| IBIS file generated by GenIBIS.pl Version 3.10
|   netra
[IBIS ver]   4.1
[File name]   DM816x.ibs
[File Rev]   1.0
[Date]   Wed Jul 14, 2010, 9:28:38
[Source]   Data created at Texas Instruments
[Notes]   Checked with IBISCHK4 : 16 warnings
   3 warnings relating to single model selectors should be waived
   13 warning relating to max data is non-monotonic should be waived
[Disclaimer] Please be aware that in the absence of a written agreement,
   Texas Instruments (TI) assumes no liability for: 1) the
   accuracy of the IBIS models provided to your company, 2) the
   proper functioning of these IBIS models in your design or for
   any resulting applications, or, 3) infringement of patents,
   copyrights, or intellectual property rights resulting from
   your use of these IBIS models. TI provides IBIS models as a
   service to our customers and therefore reserves the right to
   limit distribution of the IBIS models.
[Copyright]   Property of Texas Instruments Incorporated. Unauthorised
   reproduction and/or distribution is strictly prohibited. This
   product is protected under copyright law and trade secret law
   as an unpublished work. Created 2010,(C) Copyright 2010,
   Texas Instruments Incorporated., All Rights Reserved. These
   commodities are under the U.S. Government distribution license
   control.As such,they are not to be re-exported without the
   prior approval of the U.S. Department of Commerce.
|   Component netra
[Component]   netra
[Manufacturer]   Texas Instruments.
[Package]
|   typ   min   max
R_pkg   1083.455m   49.41m   2117.50m
L_pkg   3.26nH   0.72nH   5.80nH
C_pkg   1.9pF   0.63pF   3.17pF
[Pin]   signal_name   model_name   R_pin   L_pin   C_pin
H37   CLKIN32   Selector_1   1309.20m   3.65nH   1.83pF
F1   CLKOUT   Selector_1   1491.00m   3.78nH   1.94pF
C9   DDR0_D31   Selector_4   1469.70m   3.53nH   1.82pF
C18   DDR0_CKE   Selector_2   1358.20m   3.54nH   1.63pF
B10   DDR0_D26   Selector_4   1460.70m   3.63nH   1.97pF
D2   DDR0_D4   Selector_4   1531.00m   3.98nH   2.12pF
F2   DDR0_D1   Selector_4   1518.50m   3.74nH   2.08pF
C11   DDR0_D29   Selector_4   1449.60m   3.76nH   1.97pF
E18   DDR0_ODT0   Selector_2   1256.70m   3.57nH   1.67pF
A14   DDR0_A7   Selector_2   1331.60m   3.52nH   1.86pF
D7   DDR0_D9   Selector_4   1744.10m   4.10nH   2.16pF
C13   DDR0_CASN   Selector_2   1332.10m   3.61nH   1.86pF
C8   DDR0_D16   Selector_4   1423.40m   3.34nH   1.91pF
G10   DDR0_D28   Selector_4   1486.50m   3.61nH   2.07pF
F13   DDR0_BA0   Selector_2   1260.70m   3.24nH   1.75pF
L13   DDR0_A6   Selector_2   1153.10m   3.02nH   1.61pF
E13   DDR0_WEN   Selector_2   1287.90m   3.35nH   1.78pF
B13   DDR0_A11   Selector_2   1352.50m   3.67nH   1.95pF
D8   DDR0_D21   Selector_4   1394.50m   3.33nH   2.05pF
B12   DDR0_CLK0   Selector_2   1415.20m   3.69nH   1.69pF
C2   DDR0_DQM0   Selector_2   1527.40m   3.89nH   2.14pF
A16   DDR0_ODT1   Selector_2   1375.80m   3.74nH   1.86pF
B14   DDR0_BA1   Selector_2   1319.50m   3.63nH   1.86pF
K13   DDR0_A9   Selector_2   1252.40m   3.22nH   1.70pF
B7   DDR0_D19   Selector_4   1383.00m   3.34nH   1.95pF
B16   DDR0_A13   Selector_2   1270.10m   3.37nH   1.81pF
B6   DDR0_D13   Selector_4   1710.40m   4.12nH   2.18pF
D18   DDR0_RST   Selector_2   1315.90m   3.41nH   1.71pF
E3   DDR0_DQSN0   Selector_7   1601.30m   3.84nH   1.94pF
N14   DDR0_A8   Selector_2   1151.50m   3.06nH   1.57pF
B17   DDR0_CSN0   Selector_2   1349.40m   3.49nH   1.72pF
H10   DDR0_D18   Selector_4   1427.20m   3.35nH   2.06pF
A3   DDR0_D14   Selector_4   1766.10m   4.41nH   2.34pF
A5   DDR0_D12   Selector_4   1740.90m   4.25nH   2.37pF
A12   DDR0_CLK0N   Selector_2   1403.00m   3.48nH   1.71pF
E2   DDR0_D2   Selector_4   1529.70m   3.83nH   2.00pF
C1   DDR0_D7   Selector_4   1537.70m   3.99nH   2.06pF
N15   DDR0_BA2   Selector_2   1133.30m   3.22nH   1.44pF
B3   DDR0_D15   Selector_4   1746.20m   4.07nH   2.26pF
A9   DDR0_DQSN3   Selector_7   1585.40m   3.85nH   1.84pF
N16   DDR0_A12   Selector_2   1122.70m   3.13nH   1.44pF
C14   DDR0_A10   Selector_2   1298.30m   3.51nH   1.79pF
F3   DDR0_D6   Selector_4   1543.60m   4.02nH   2.09pF
B2   DDR0_D5   Selector_4   1489.90m   3.72nH   2.04pF
A8   DDR0_DQSN2   Selector_7   1538.30m   3.73nH   1.90pF
B9   DDR0_DQS3   Selector_7   1600.40m   3.82nH   1.84pF
B5   DDR0_DQM1   Selector_2   1739.40m   4.39nH   2.24pF
E8   DDR0_D27   Selector_4   1430.00m   3.59nH   1.99pF
J11   DDR0_D30   Selector_4   1504.00m   3.69nH   1.90pF
J13   DDR0_A5   Selector_2   1333.50m   3.39nH   1.68pF
E7   DDR0_D23   Selector_4   1403.30m   3.52nH   1.96pF
A13   DDR0_A0   Selector_2   1265.50m   3.65nH   1.74pF
A15   DDR0_CLK1   Selector_2   1409.10m   3.47nH   1.71pF
A4   DDR0_DQSN1   Selector_7   1881.10m   4.39nH   2.13pF
G4   DDR0_D3   Selector_4   1490.40m   3.74nH   2.07pF
B8   DDR0_DQS2   Selector_7   1535.10m   3.81nH   1.76pF
A7   DDR0_D17   Selector_4   1476.50m   3.78nH   1.93pF
B4   DDR0_DQS1   Selector_7   1878.40m   4.27nH   2.13pF
D17   DDR0_A14   Selector_2   1253.70m   3.19nH   1.81pF
C6   DDR0_D10   Selector_4   1782.00m   4.37nH   2.22pF
H13   DDR0_A4   Selector_2   1256.10m   3.18nH   1.74pF
E9   DDR0_D24   Selector_4   1434.50m   3.63nH   1.86pF
D9   DDR0_DQM3   Selector_2   1479.60m   3.74nH   1.92pF
D13   DDR0_RASN   Selector_2   1266.70m   3.18nH   1.82pF
B1   DDR0_D0   Selector_4   1470.70m   3.76nH   2.13pF
C5   DDR0_D8   Selector_4   1688.70m   3.78nH   2.09pF
N17   DDR0_A1   Selector_2   1196.40m   3.20nH   1.58pF
F8   DDR0_D20   Selector_4   1427.80m   3.64nH   1.98pF
F9   DDR0_D22   Selector_4   1439.50m   3.61nH   1.90pF
D6   DDR0_D11   Selector_4   1736.00m   3.98nH   2.27pF
G9   DDR0_DQM2   Selector_2   1448.90m   3.58nH   1.95pF
F4   DDR0_DQS0   Selector_7   1620.50m   3.95nH   1.97pF
F18   DDR0_CSN1   Selector_2   1308.20m   3.34nH   1.73pF
D15   DDR0_A2   Selector_2   1293.60m   3.44nH   1.80pF
G13   DDR0_A3   Selector_2   1313.50m   3.47nH   1.69pF
B15   DDR0_CLK1N   Selector_2   1400.90m   3.42nH   1.71pF
B11   DDR0_D25   Selector_4   1487.80m   3.56nH   1.92pF
F36   DDR1_D1   Selector_4   1516.50m   3.72nH   2.10pF
K25   DDR1_A9   Selector_2   1252.70m   3.22nH   1.71pF
B27   DDR1_D25   Selector_4   1494.60m   3.90nH   1.92pF
A35   DDR1_D14   Selector_4   1761.50m   4.48nH   2.31pF
E35   DDR1_DQSN0   Selector_7   1600.60m   3.84nH   1.86pF
L25   DDR1_A6   Selector_2   1146.20m   2.92nH   1.59pF
G34   DDR1_D3   Selector_4   1489.80m   3.78nH   2.08pF
B32   DDR1_D13   Selector_4   1708.80m   4.35nH   2.32pF
C20   DDR1_CKE   Selector_2   1327.50m   3.43nH   1.63pF
C24   DDR1_A10   Selector_2   1281.10m   3.40nH   1.81pF
D20   DDR1_RST   Selector_2   1302.90m   3.49nH   1.67pF
C29   DDR1_D31   Selector_4   1476.80m   3.76nH   1.94pF
E29   DDR1_D24   Selector_4   1437.50m   3.70nH   1.97pF
B22   DDR1_A13   Selector_2   1250.70m   3.43nH   1.78pF
C33   DDR1_D8   Selector_4   1686.90m   4.14nH   2.13pF
B31   DDR1_D19   Selector_4   1383.90m   3.59nH   1.84pF
C37   DDR1_D7   Selector_4   1538.40m   3.97nH   2.11pF
B33   DDR1_DQM1   Selector_2   1739.30m   4.30nH   2.28pF
E36   DDR1_D2   Selector_4   1529.70m   3.92nH   2.08pF
F20   DDR1_CSN1   Selector_2   1298.80m   3.39nH   1.72pF
D25   DDR1_RASN   Selector_2   1251.90m   3.31nH   1.80pF
C36   DDR1_DQM0   Selector_2   1526.50m   4.01nH   2.09pF
N22   DDR1_A12   Selector_2   1129.60m   3.36nH   1.44pF
N24   DDR1_A8   Selector_2   1151.30m   3.03nH   1.54pF
B21   DDR1_CSN0   Selector_2   1338.00m   3.57nH   1.74pF
B36   DDR1_D5   Selector_4   1496.60m   3.79nH   2.09pF
N21   DDR1_A1   Selector_2   1193.70m   3.19nH   1.60pF
F30   DDR1_D20   Selector_4   1426.70m   3.75nH   1.94pF
E30   DDR1_D27   Selector_4   1425.40m   3.68nH   2.08pF
C30   DDR1_D16   Selector_4   1420.60m   3.50nH   2.00pF
A34   DDR1_DQSN1   Selector_7   1885.10m   4.38nH   2.14pF
B28   DDR1_D26   Selector_4   1457.10m   3.72nH   1.90pF
A25   DDR1_A0   Selector_2   1266.80m   3.73nH   1.79pF
J27   DDR1_D30   Selector_4   1507.60m   3.72nH   2.06pF
A26   DDR1_CLK0N   Selector_2   1408.90m   3.58nH   1.67pF
B37   DDR1_D0   Selector_4   1469.70m   3.83nH   2.00pF
F35   DDR1_D6   Selector_4   1543.90m   3.99nH   2.08pF
N23   DDR1_BA2   Selector_2   1141.30m   3.31nH   1.43pF
B26   DDR1_CLK0   Selector_2   1421.50m   3.73nH   1.56pF
E20   DDR1_ODT0   Selector_2   1246.60m   3.51nH   1.69pF
B25   DDR1_A11   Selector_2   1335.80m   3.85nH   1.84pF
D21   DDR1_A14   Selector_2   1262.30m   3.15nH   1.77pF
B30   DDR1_DQS2   Selector_7   1543.40m   3.74nH   1.70pF
A31   DDR1_D17   Selector_4   1477.60m   3.79nH   1.89pF
E31   DDR1_D23   Selector_4   1404.30m   3.60nH   2.03pF
C27   DDR1_D29   Selector_4   1448.30m   3.80nH   2.01pF
A29   DDR1_DQSN3   Selector_7   1598.60m   3.83nH   1.94pF
J25   DDR1_A5   Selector_2   1309.60m   3.41nH   1.73pF
G29   DDR1_DQM2   Selector_2   1449.00m   3.60nH   1.92pF
D29   DDR1_DQM3   Selector_2   1482.20m   3.81nH   2.01pF
C25   DDR1_CASN   Selector_2   1319.50m   3.60nH   1.85pF
A22   DDR1_ODT1   Selector_2   1360.60m   3.61nH   1.87pF
E25   DDR1_WEN   Selector_2   1267.60m   3.39nH   1.80pF
A30   DDR1_DQSN2   Selector_7   1544.90m   3.83nH   1.76pF
D32   DDR1_D11   Selector_4   1733.00m   4.16nH   2.21pF
F34   DDR1_DQS0   Selector_7   1622.30m   3.89nH   1.76pF
B29   DDR1_DQS3   Selector_7   1607.10m   4.02nH   1.86pF
A33   DDR1_D12   Selector_4   1736.90m   4.33nH   2.28pF
D31   DDR1_D9   Selector_4   1747.90m   4.19nH   2.19pF
A24   DDR1_A7   Selector_2   1317.50m   3.61nH   1.88pF
H25   DDR1_A4   Selector_2   1241.80m   3.15nH   1.69pF
G28   DDR1_D28   Selector_4   1477.50m   3.63nH   2.05pF
D36   DDR1_D4   Selector_4   1532.20m   3.94nH   2.16pF
G25   DDR1_A3   Selector_2   1301.50m   3.47nH   1.74pF
B24   DDR1_BA1   Selector_2   1300.70m   3.55nH   1.82pF
D30   DDR1_D21   Selector_4   1394.40m   3.59nH   1.98pF
D23   DDR1_A2   Selector_2   1279.00m   3.38nH   1.87pF
F25   DDR1_BA0   Selector_2   1249.40m   3.21nH   1.71pF
H28   DDR1_D18   Selector_4   1427.50m   3.48nH   1.90pF
B35   DDR1_D15   Selector_4   1754.70m   4.28nH   2.24pF
F29   DDR1_D22   Selector_4   1441.70m   3.68nH   1.89pF
A23   DDR1_CLK1   Selector_2   1408.60m   3.54nH   1.77pF
C32   DDR1_D10   Selector_4   1784.80m   4.48nH   2.18pF
B34   DDR1_DQS1   Selector_7   1881.40m   4.41nH   2.08pF
B23   DDR1_CLK1N   Selector_2   1400.10m   3.58nH   1.69pF
J35   EMU0   Selector_3   1645.80m   4.47nH   2.22pF
L36   EMU1   Selector_3   1287.90m   3.82nH   1.76pF
L37   EMU2   Selector_3   1334.20m   3.65nH   1.85pF
M36   EMU3   Selector_3   1079.80m   3.03nH   1.65pF
M37   EMU4   Selector_3   1302.60m   3.45nH   1.77pF
AG28   GMII0_TXD4   Selector_3   564.85m   1.69nH   1.08pF
AE34   GMII0_RXER   Selector_3   916.91m   2.56nH   1.42pF
AF36   GMII0_TXD5   Selector_3   1240.00m   3.21nH   1.63pF
AF37   GMII0_TXCLK   Selector_3   1350.00m   3.67nH   1.87pF
AD25   GMII0_RXD5   Selector_3   170.60m   1.01nH   0.78pF
AE36   GMII0_RXD7   Selector_3   1288.30m   3.53nH   1.68pF
AE30   GMII0_TXD3   Selector_3   493.69m   1.61nH   1.01pF
AE33   GMII0_TXD0   Selector_3   986.48m   2.66nH   1.40pF
AE37   GMII0_RXCLK   Selector_3   1509.90m   3.89nH   2.04pF
AE32   GMII0_TXD1   Selector_3   762.14m   2.22nH   1.20pF
AG35   GMII0_TXD7   Selector_3   1051.50m   2.91nH   1.59pF
AC35   GMII0_RXD4   Selector_3   1124.40m   3.09nH   1.69pF
AC25   GMII0_RXD6   Selector_3   92.81m   0.81nH   0.65pF
AE31   GMII0_TXD2   Selector_3   828.93m   2.29nH   1.22pF
AG36   GMII0_TXD6   Selector_3   1331.80m   3.61nH   1.78pF
AD35   GMII0_RXD3   Selector_3   947.25m   2.61nH   1.46pF
AD37   GMII0_RXD0   Selector_3   1306.50m   3.47nH   1.77pF
AD36   GMII0_RXD1   Selector_3   1427.60m   3.90nH   1.76pF
AA25   GMII0_CRS   Selector_3   100.59m   0.85nH   0.71pF
AC37   GMII0_GTXCLK   Selector_3   1221.60m   3.13nH   1.69pF
AG37   GMII0_TXEN   Selector_3   1452.10m   3.88nH   1.95pF
AB25   GMII0_COL   Selector_3   226.60m   1.06nH   0.71pF
AE35   GMII0_RXDV   Selector_3   1056.10m   2.91nH   1.55pF
AC36   GMII0_RXD2   Selector_3   1200.10m   3.19nH   1.70pF
K31   GP0_IO0   Selector_1   795.97m   2.24nH   1.35pF
G5   GP0_IO6   Selector_1   1196.30m   3.27nH   1.74pF
G2   GP0_IO5   Selector_1   1205.80m   3.58nH   1.79pF
H32   GP0_IO4   Selector_1   1092.10m   2.82nH   1.67pF
H35   GP0_IO7   Selector_1   1083.40m   3.13nH   1.75pF
K30   GP0_IO2   Selector_1   925.22m   2.65nH   1.41pF
L29   GP0_IO1   Selector_1   694.30m   2.11nH   1.26pF
J31   GP0_IO3   Selector_1   1017.90m   2.83nH   1.55pF
J33   GP1_IO31   Selector_1   1137.80m   3.33nH   1.68pF
J32   GP1_IO30   Selector_1   1020.50m   2.79nH   1.56pF
AA3   GPMC_D3   Selector_1   1056.40m   2.99nH   1.56pF
AE1   GPMC_A4   Selector_1   1377.50m   3.92nH   1.90pF
AD3   GPMC_A7   Selector_1   1196.70m   3.32nH   1.73pF
W3   GPMC_D10   Selector_1   1112.50m   3.04nH   1.53pF
Y10   GPMC_D6   Selector_1   352.48m   1.25nH   0.89pF
AD1   GPMC_A10   Selector_1   1395.90m   3.72nH   1.87pF
Y3   GPMC_D4   Selector_1   1143.00m   3.16nH   1.62pF
AD8   GPMC_A6   Selector_1   1530.30m   4.11nH   2.05pF
AG3   GPMC_CS4   Selector_1   1297.50m   3.69nH   1.80pF
W2   GPMC_D12   Selector_1   966.20m   2.79nH   1.53pF
AC2   GPMC_A11   Selector_1   1362.40m   3.66nH   1.85pF
AC1   GPMC_D0   Selector_1   1233.50m   3.39nH   1.85pF
AA2   GPMC_D5   Selector_1   1118.40m   3.28nH   1.58pF
AE2   GPMC_A5   Selector_1   1495.60m   3.99nH   1.96pF
V1   GPMC_CLK   Selector_1   1272.40m   3.48nH   1.79pF
AG2   GPMC_WEN   Selector_1   1545.10m   4.10nH   2.08pF
V10   GPMC_D13   Selector_1   184.75m   0.89nH   0.73pF
AE4   GPMC_A2   Selector_1   1235.40m   3.43nH   1.67pF
AA4   GPMC_D1   Selector_1   1051.20m   2.95nH   1.51pF
AH7   GPMC_CS0   Selector_1   1189.60m   3.37nH   1.71pF
Y1   GPMC_D9   Selector_1   1157.00m   3.26nH   1.75pF
AH1   GPMC_CS1   Selector_1   1653.70m   4.70nH   2.01pF
AE10   GPMC_ADVN_ALE   Selector_1   1720.10m   4.77nH   2.21pF
AD4   GPMC_A8   Selector_1   1152.80m   3.26nH   1.73pF
AE7   GPMC_DIR   Selector_1   1320.10m   3.72nH   1.87pF
AE3   GPMC_A3   Selector_1   1358.60m   3.79nH   1.85pF
AF2   GPMC_OEN_REN   Selector_1   1476.20m   3.88nH   1.94pF
AH2   GPMC_CS2   Selector_1   1411.50m   3.83nH   2.11pF
AG1   GPMC_CS5   Selector_1   1663.40m   4.38nH   2.09pF
Y2   GPMC_D7   Selector_1   1171.80m   3.24nH   1.63pF
W1   GPMC_D11   Selector_1   1141.60m   3.23nH   1.64pF
W4   GPMC_D8   Selector_1   980.65m   2.85nH   1.47pF
AE11   GPMC_BE0N_CLE   Selector_1   532.49m   1.84nH   1.17pF
V2   GPMC_D15   Selector_1   1141.50m   3.10nH   1.63pF
AF1   GPMC_BE1N   Selector_1   1416.40m   3.85nH   2.00pF
AD2   GPMC_A9   Selector_1   1429.00m   3.83nH   1.94pF
AE9   GPMC_WPN   Selector_1   1318.70m   3.47nH   1.88pF
AE6   GPMC_A0   Selector_1   1350.00m   3.73nH   2.00pF
V3   GPMC_D14   Selector_1   1008.30m   2.79nH   1.47pF
AG9   GPMC_CS3   Selector_1   1366.30m   3.85nH   2.05pF
AC5   GPMC_A27   Selector_1   1270.00m   3.50nH   1.93pF
AE8   GPMC_WAIT   Selector_1   1441.30m   4.00nH   1.90pF
AB2   GPMC_D2   Selector_1   1290.40m   3.51nH   1.73pF
AE5   GPMC_A1   Selector_1   1097.80m   3.10nH   1.66pF
AE24   HDMI_HPDET   Selector_1   316.48m   1.39nH   0.87pF
AP25   HDMI_CEC   Selector_1   1161.80m   3.19nH   1.63pF
AL25   HDMI_SCL   Selector_5   1122.30m   3.12nH   1.65pF
AK25   HDMI_SDA   Selector_5   1029.40m   2.70nH   1.63pF
N33   IIC0_SDA   Selector_5   750.94m   2.35nH   1.20pF
N32   IIC0_SCL   Selector_5   612.69m   1.99nH   1.17pF
N35   IIC1_SDA   Selector_5   1136.40m   3.15nH   1.69pF
N34   IIC1_SCL   Selector_5   975.35m   2.79nH   1.48pF
AJ32   MCA0_AXR1   Selector_1   1267.10m   3.43nH   1.71pF
AJ36   MCA0_AXR4   Selector_1   1321.90m   3.59nH   1.93pF
AG29   MCA0_AFSR   Selector_1   574.77m   1.74nH   1.06pF
AJ31   MCA0_AFSX   Selector_1   946.20m   2.58nH   1.39pF
AH31   MCA0_ACLKHX   Selector_1   808.09m   2.43nH   1.29pF
AK37   MCA0_AXR0   Selector_1   1454.10m   3.84nH   1.91pF
AJ27   MCA0_AHCLKR   Selector_1   528.21m   1.54nH   1.02pF
AJ37   MCA0_AXR5   Selector_1   1303.30m   3.38nH   1.90pF
AJ33   MCA0_AXR2   Selector_1   1310.90m   3.50nH   1.79pF
AJ35   MCA0_AMUTE   Selector_1   1238.10m   3.28nH   1.65pF
AJ34   MCA0_AXR3   Selector_1   1356.50m   3.64nH   1.82pF
AK28   MCA0_ACLKR   Selector_1   691.13m   2.17nH   1.19pF
AH30   MCA0_ACLKX   Selector_1   727.97m   2.17nH   1.16pF
AK36   MCA1_ACLKR   Selector_1   1296.00m   3.73nH   1.90pF
AK32   MCA1_AXR1   Selector_1   1015.70m   2.72nH   1.48pF
AK34   MCA1_AFSX   Selector_1   1182.80m   3.36nH   1.76pF
AL33   MCA1_AXR0   Selector_1   1175.20m   3.24nH   1.75pF
AK35   MCA1_AFSR   Selector_1   1404.40m   3.71nH   2.00pF
AL36   MCA1_ACLKX   Selector_1   1648.10m   4.37nH   2.19pF
AM37   MCA1_ACLKHX   Selector_1   1557.70m   4.14nH   2.05pF
AK33   MCA1_AMUTE   Selector_1   1127.60m   2.94nH   1.66pF
AL37   MCA1_AHCLKR   Selector_1   1549.50m   4.00nH   2.09pF
AM36   MCA2_ACLKX   Selector_1   1446.70m   4.09nH   1.93pF
AM35   MCA2_AFSR   Selector_1   1487.90m   4.07nH   1.90pF
AN36   MCA2_ACLKHX   Selector_1   1652.90m   4.24nH   2.15pF
AL34   MCA2_ACLKR   Selector_1   1200.30m   3.13nH   1.75pF
AR36   MCA2_AXR0   Selector_1   1739.00m   4.42nH   2.24pF
AN35   MCA2_AFSX   Selector_1   1404.00m   3.87nH   2.02pF
AP36   MCA2_AMUTE   Selector_1   1538.80m   4.58nH   2.10pF
AR37   MCA2_AXR1   Selector_1   1784.60m   4.90nH   2.34pF
AM34   MCA2_AHCLKR   Selector_1   1381.00m   3.66nH   1.84pF
AR29   MCARD_VCCEN   Selector_1   1416.30m   3.63nH   1.90pF
AT28   MCARD_RESET   Selector_1   1200.10m   3.31nH   1.74pF
AN29   MCARD_VS1   Selector_1   1177.60m   3.06nH   1.62pF
AP29   MCARD_VS2   Selector_1   1198.90m   3.48nH   1.75pF
AL28   MCARD_CD1   Selector_1   999.58m   2.85nH   1.59pF
AM29   MCARD_MDET   Selector_1   1260.30m   3.63nH   1.76pF
AT29   MCARD_VPPEN   Selector_1   1429.70m   4.08nH   1.87pF
AL29   MCARD_CD2   Selector_1   1165.90m   3.32nH   1.56pF
AR30   MCTL_SCTL   Selector_3   1353.40m   3.90nH   1.89pF
AN31   MCTL_SDI   Selector_3   1339.00m   3.72nH   1.83pF
AT30   MCTL_SCLK   Selector_3   1568.10m   4.28nH   2.08pF
AN30   MCTL_SDO   Selector_3   1352.10m   3.58nH   1.79pF
AH37   MDIO_MCLK   Selector_1   1273.70m   3.46nH   1.85pF
AH36   MDIO_MDIO   Selector_1   1172.50m   3.05nH   1.63pF
U2   MMC_CLK   Selector_1   975.81m   2.83nH   1.48pF
T2   MMC_DAT2_SDRW   Selector_1   1149.00m   3.23nH   1.66pF
U4   MMC_POW   Selector_1   829.64m   2.47nH   1.30pF
U3   MMC_CMD   Selector_1   992.29m   2.99nH   1.45pF
T1   MMC_DAT1_SDIRQ   Selector_1   1078.00m   3.08nH   1.60pF
R13   MMC_SDCD   Selector_1   221.26m   1.25nH   0.82pF
T13   MMC_DAT3   Selector_1   271.80m   1.19nH   0.84pF
U1   MMC_DAT0   Selector_1   1206.20m   3.39nH   1.68pF
R5   MMC_SDWP   Selector_1   904.81m   2.64nH   1.32pF
AT36   MTSI_DATA0   Selector_3   1623.80m   4.40nH   2.14pF
AU34   MTSI_DATA6   Selector_3   1858.20m   5.09nH   2.51pF
AT34   MTSI_DATA3   Selector_3   1793.70m   4.65nH   2.21pF
AT33   MTSI_BYTSTRT   Selector_3   1519.30m   4.11nH   2.10pF
AR33   MTSI_DATA5   Selector_3   1589.90m   4.08nH   2.09pF
AU36   MTSI_DATA2   Selector_3   1943.20m   4.97nH   2.40pF
AT37   MTSI_DCLK   Selector_3   1743.20m   4.77nH   2.32pF
AT35   MTSI_DATA1   Selector_3   1674.40m   4.57nH   2.13pF
AP32   MTSI_DATA7   Selector_3   1347.40m   3.62nH   1.88pF
AU35   MTSI_DATA4   Selector_3   1865.90m   4.74nH   2.42pF
AT31   MTSO_DATA5   Selector_3   1489.10m   4.26nH   1.93pF
AU30   MTSO_BYTSTRT   Selector_3   1493.30m   4.07nH   2.01pF
AP30   MTSO_DATA6   Selector_3   1528.60m   4.24nH   1.97pF
AM30   MTSO_DATA7   Selector_3   1204.30m   3.33nH   1.65pF
AR32   MTSO_DATA1   Selector_3   1395.10m   3.95nH   1.95pF
AU33   MTSO_DCLK   Selector_3   1708.70m   4.59nH   2.17pF
AT32   MTSO_DATA2   Selector_3   1667.80m   4.59nH   2.05pF
AU32   MTSO_DATA3   Selector_3   1538.00m   4.30nH   2.17pF
AU31   MTSO_DATA4   Selector_3   1696.40m   4.60nH   2.24pF
AP31   MTSO_DATA0   Selector_3   1401.40m   3.88nH   1.91pF
G36   NMIN   Selector_1   1218.30m   3.39nH   1.76pF
F37   PORZ   Selector_9   1487.00m   3.97nH   1.84pF
G33   RESETN   Selector_1   1164.50m   3.18nH   1.65pF
G37   RSTOUTN   Selector_1   1491.30m   4.03nH   2.05pF
J36   RTCK   Selector_1   1441.60m   3.91nH   1.92pF
J4   SC0_VCCEN   Selector_1   1051.60m   2.94nH   1.64pF
J7   SC0_DATA   Selector_1   1173.20m   3.20nH   1.70pF
K2   SC0_RST   Selector_1   1115.70m   3.16nH   1.71pF
K8   SC0_DET   Selector_1   879.20m   2.55nH   1.43pF
J5   SC0_C4   Selector_1   1061.30m   3.17nH   1.63pF
J3   SC0_VPPEN   Selector_1   1308.40m   3.54nH   1.75pF
J6   SC0_CLK   Selector_1   1225.70m   3.47nH   1.74pF
H6   SC1_DATA   Selector_1   1045.70m   3.38nH   1.56pF
H2   SC1_VPPEN   Selector_1   1117.60m   3.22nH   1.57pF
J1   SC1_RST   Selector_1   1395.10m   3.87nH   1.92pF
H5   SC1_CLK   Selector_1   1173.60m   3.57nH   1.70pF
H4   SC1_C4   Selector_1   1249.30m   3.40nH   1.66pF
J2   SC1_DET   Selector_1   1182.70m   3.29nH   1.76pF
H3   SC1_VCCEN   Selector_1   1193.00m   3.32nH   1.78pF
R2   SPI_SCLK   Selector_1   1165.00m   3.30nH   1.69pF
N11   SPI_D0   Selector_1   510.79m   1.68nH   1.05pF
P3   SPI_SCS2   Selector_1   987.83m   2.80nH   1.53pF
P1   SPI_SCS3   Selector_1   1096.00m   3.15nH   1.70pF
P13   SPI_D1   Selector_1   145.99m   0.87nH   0.73pF
R1   SPI_SCS0   Selector_1   1135.00m   3.30nH   1.57pF
P2   SPI_SCS1   Selector_1   1213.40m   3.45nH   1.69pF
J37   TCLK   Selector_8   1317.20m   3.79nH   1.87pF
J34   TDI   Selector_8   1591.40m   4.51nH   2.12pF
N30   TDO   Selector_3   623.22m   1.99nH   1.23pF
H33   TIM4_OUT   Selector_1   1137.00m   3.34nH   1.66pF
H34   TIM5_OUT   Selector_1   1275.80m   3.46nH   1.79pF
H1   TIM6_OUT   Selector_1   1253.50m   3.62nH   1.76pF
G1   TIM7_OUT   Selector_1   1398.80m   4.13nH   1.83pF
N31   TMS   Selector_1   700.89m   2.16nH   1.32pF
K36   TRSTN   Selector_8   1293.50m   3.74nH   1.76pF
AR1   TSI0_PACERR   Selector_3   1802.10m   5.00nH   2.40pF
AT1   TSI0_PACVAL   Selector_3   1979.70m   5.80nH   2.46pF
AP2   TSI0_DCLK   Selector_3   1694.20m   4.68nH   2.23pF
AU3   TSI0_DATA   Selector_3   2117.50m   5.77nH   2.72pF
AN2   TSI0_BYTSTRT   Selector_3   1543.30m   4.17nH   2.20pF
AN7   TSI1_DATA   Selector_3   1213.20m   3.57nH   1.77pF
AD13   TSI1_PACERR   Selector_3   104.10m   0.86nH   0.69pF
AP8   TSI1_BYTSTRT   Selector_3   1276.80m   3.77nH   1.72pF
AM8   TSI1_DCLK   Selector_3   955.08m   2.77nH   1.46pF
AN8   TSI1_PACVAL   Selector_3   1361.20m   3.75nH   1.84pF
AU4   TSI2_BYTSTRT   Selector_3   2068.40m   5.19nH   2.61pF
AM3   TSI2_DCLK   Selector_3   1486.90m   4.13nH   2.13pF
AR2   TSI2_PACVAL   Selector_3   1623.10m   4.50nH   2.18pF
AT2   TSI2_PACERR   Selector_3   1749.50m   4.88nH   2.30pF
AN3   TSI2_DATA   Selector_3   1465.70m   4.13nH   2.11pF
AK6   TSI3_PACERR   Selector_3   988.10m   2.94nH   1.48pF
AR6   TSI3_DATA   Selector_3   1381.20m   3.80nH   1.90pF
AC13   TSI3_DCLK   Selector_3   155.01m   1.03nH   0.72pF
AP6   TSI3_PACVAL   Selector_3   1445.20m   4.18nH   1.89pF
AT6   TSI3_BYTSTRT   Selector_3   1571.00m   4.35nH   2.16pF
AK5   TSI4_PACVAL   Selector_3   1069.10m   3.00nH   1.67pF
AK4   TSI4_PACERR   Selector_3   1433.00m   4.30nH   2.02pF
AL5   TSI4_BYTSTRT   Selector_3   1078.00m   3.24nH   1.61pF
AR5   TSI4_DCLK   Selector_3   1614.20m   4.48nH   2.10pF
AT5   TSI4_DATA   Selector_3   1629.60m   4.24nH   2.16pF
AR9   TSI5_DATA   Selector_3   1366.30m   3.49nH   1.73pF
AU8   TSI5_PACERR   Selector_3   1507.00m   3.98nH   1.89pF
AP9   TSI5_PACVAL   Selector_3   1029.30m   3.03nH   1.48pF
AT9   TSI5_BYTSTRT   Selector_3   1193.10m   3.31nH   1.65pF
AJ11   TSI5_DCLK   Selector_3   549.21m   1.80nH   1.00pF
AL4   TSI6_PACVAL   Selector_3   1190.50m   3.43nH   1.71pF
AU5   TSI6_DATA   Selector_3   1870.90m   4.92nH   2.39pF
AM4   TSI6_BYTSTRT   Selector_3   1322.30m   3.61nH   1.91pF
AT4   TSI6_DCLK   Selector_3   1755.50m   4.94nH   2.26pF
AT3   TSI6_PACERR   Selector_3   1774.10m   4.84nH   2.32pF
AR8   TSI7_PACVAL   Selector_3   1291.70m   3.62nH   1.76pF
AT8   TSI7_PACERR   Selector_3   1280.60m   3.58nH   1.81pF
AL9   TSI7_BYTSTRT   Selector_3   961.15m   2.67nH   1.40pF
AN9   TSI7_DATA   Selector_3   1032.00m   2.99nH   1.55pF
AM9   TSI7_DCLK   Selector_3   1053.70m   2.93nH   1.49pF
AP1   TSO0_DCLK   Selector_3   1650.20m   4.42nH   2.28pF
AM2   TSO0_DATA   Selector_3   1471.90m   4.29nH   2.02pF
AL2   TSO0_BYTSTRT   Selector_3   1458.20m   4.17nH   2.00pF
AL1   TSO0_PACERR   Selector_3   1673.30m   4.64nH   2.18pF
AK1   TSO0_PACVAL   Selector_3   1622.70m   4.67nH   2.10pF
AU6   TSO1_PACVAL   Selector_3   1546.80m   4.48nH   2.10pF
AU7   TSO1_DATA   Selector_3   1606.70m   4.46nH   2.06pF
AP7   TSO1_BYTSTRT   Selector_3   1378.80m   3.95nH   1.76pF
AJ7   TSO1_PACERR   Selector_3   1044.50m   3.12nH   1.54pF
AT7   TSO1_DCLK   Selector_3   1406.70m   3.83nH   2.00pF
N8   UART0_TXD   Selector_1   868.60m   2.50nH   1.32pF
N10   UART0_RXD   Selector_1   748.15m   2.28nH   1.19pF
N7   UART0_CTSN   Selector_1   705.88m   2.28nH   1.24pF
N5   UART0_DCDN   Selector_1   827.57m   2.44nH   1.40pF
N9   UART0_RTSN   Selector_1   628.93m   1.93nH   1.12pF
N6   UART0_DTRN   Selector_1   922.02m   2.79nH   1.39pF
N4   UART0_DSRN   Selector_1   994.06m   2.84nH   1.50pF
N3   UART0_RIN   Selector_1   1130.30m   3.18nH   1.60pF
L3   UART1_CTSN   Selector_1   1169.80m   3.36nH   1.60pF
M2   UART1_RTSN   Selector_1   1056.30m   3.10nH   1.76pF
N2   UART1_TXD   Selector_1   1125.70m   3.22nH   1.54pF
N1   UART1_RXD   Selector_1   1089.60m   3.17nH   1.69pF
K7   UART2_CTSN   Selector_1   945.39m   2.78nH   1.51pF
M1   UART2_RXD   Selector_1   1382.50m   3.76nH   1.92pF
L2   UART2_TXD   Selector_1   1115.30m   3.17nH   1.66pF
L9   UART2_RTSN   Selector_1   842.24m   2.44nH   1.23pF
P35   USB0_DRVVBUS   Selector_6   1089.00m   3.00nH   1.60pF
R35   USB1_DRVVBUS   Selector_6   979.53m   2.82nH   1.54pF
AR18   VIN0_D3   Selector_3   1492.40m   4.06nH   1.92pF
AP17   VIN0_D8   Selector_3   1257.20m   3.41nH   1.78pF
AE16   VIN0_D9   Selector_3   131.92m   0.96nH   0.74pF
AU15   VIN0_D14   Selector_3   1374.00m   3.75nH   1.78pF
AR14   VIN0_CLK0   Selector_3   1177.50m   3.33nH   1.81pF
AU14   VIN0_D15   Selector_3   1352.60m   3.58nH   1.84pF
AU17   VIN0_D11   Selector_3   1491.10m   4.08nH   1.87pF
AT18   VIN0_D4   Selector_3   1510.80m   4.01nH   1.96pF
AU16   VIN0_D12   Selector_3   1315.80m   3.94nH   1.86pF
AH18   VIN0_D2   Selector_3   872.75m   2.31nH   1.32pF
AT16   VIN0_D10   Selector_3   1230.30m   3.72nH   1.71pF
AR19   VIN0_CLK1   Selector_3   1341.60m   3.64nH   1.82pF
AP18   VIN0_D6   Selector_3   1420.70m   3.57nH   1.86pF
AU18   VIN0_D1   Selector_3   1358.60m   3.72nH   1.93pF
AR17   VIN0_D7   Selector_3   1254.10m   3.52nH   1.68pF
AT15   VIN0_D13   Selector_3   1198.30m   3.34nH   1.74pF
AT17   VIN0_D5   Selector_3   1241.40m   3.52nH   1.84pF
AJ19   VIN0_D0   Selector_3   1023.40m   2.63nH   1.45pF
AK2   VLYNQ_SCRUN   Selector_3   1410.60m   3.93nH   1.94pF
AJ2   VLYNQ_TXD2   Selector_3   1514.70m   4.21nH   2.05pF
AH8   VLYNQ_TXD3   Selector_3   1099.90m   3.07nH   1.58pF
AJ4   VLYNQ_RXD3   Selector_3   1241.90m   3.63nH   1.87pF
AJ1   VLYNQ_CLOCK   Selector_3   1624.10m   4.48nH   2.15pF
AJ3   VLYNQ_TXD0   Selector_3   1462.40m   4.01nH   1.99pF
AJ6   VLYNQ_RXD1   Selector_3   1343.60m   3.71nH   1.89pF
AB13   VLYNQ_RXD0   Selector_3   160.17m   0.98nH   0.78pF
AK3   VLYNQ_TXD1   Selector_3   1529.30m   4.11nH   2.10pF
AJ5   VLYNQ_RXD2   Selector_3   1264.90m   3.50nH   1.90pF
AG13   VOUT0_R_CR4   Selector_3   217.78m   1.00nH   0.73pF
AL13   VOUT0_B_CB_C3   Selector_3   690.20m   2.13nH   1.17pF
AT11   VOUT0_R_CR2   Selector_3   1157.90m   3.04nH   1.60pF
AR11   VOUT0_R_CR3   Selector_3   1204.20m   3.21nH   1.49pF
AE14   VOUT0_G_Y_YC6   Selector_3   49.41m   0.72nH   0.63pF
AP14   VOUT0_G_Y_YC3   Selector_3   1087.90m   2.97nH   1.55pF
AU9   VOUT0_R_CR9   Selector_3   1537.60m   3.98nH   1.92pF
AT10   VOUT0_R_CR5   Selector_3   1370.10m   3.64nH   1.73pF
AR13   VOUT0_G_Y_YC9   Selector_3   1023.70m   2.96nH   1.49pF
AL14   VOUT0_G_Y_YC4   Selector_3   1234.60m   3.55nH   1.77pF
AP13   VOUT0_B_CB_C2   Selector_3   917.76m   2.65nH   1.36pF
AT14   VOUT0_CLK   Selector_3   1310.60m   3.66nH   1.77pF
AE15   VOUT0_G_Y_YC2   Selector_3   151.06m   0.89nH   0.76pF
AK10   VOUT0_R_CR8   Selector_3   781.57m   2.22nH   1.14pF
AU10   VOUT0_R_CR6   Selector_3   1382.50m   3.58nH   1.80pF
AT12   VOUT0_B_CB_C9   Selector_3   1085.10m   2.92nH   1.62pF
AM14   VOUT0_G_Y_YC5   Selector_3   968.59m   2.74nH   1.44pF
AK13   VOUT0_B_CB_C5   Selector_3   665.88m   2.05nH   1.13pF
AU13   VOUT0_G_Y_YC8   Selector_3   1388.60m   4.10nH   1.72pF
AN13   VOUT0_B_CB_C4   Selector_3   863.96m   2.52nH   1.28pF
AJ13   VOUT0_B_CB_C6   Selector_3   548.25m   1.76nH   1.05pF
AM13   VOUT0_B_CB_C7   Selector_3   856.98m   2.52nH   1.28pF
AH13   VOUT0_B_CB_C8   Selector_3   489.34m   1.53nH   0.94pF
AT13   VOUT0_G_Y_YC7   Selector_3   1050.90m   3.01nH   1.60pF
AL10   VOUT0_R_CR7   Selector_3   789.95m   2.20nH   1.14pF
H36   WD_OUT   Selector_1   1132.30m   3.29nH   1.67pF
| Device pads which are not required to be modeled. Included for completeness
|D14   AMUX_DDR_PLL   BFTHRUDDG_WRP.PAD
|AUTO2   AMUX_AUDIO_PLL   BFTHRUDDG_WRP.PAD
|D24   AMUX_MAIN_PLL   BFTHRUDDG_WRP.PAD
|AUTO1   AMUX_VIDEO_PLL   BFTHRUDDG_WRP.PAD
|A6   DDR0_VTP   OVTPOSHTLTCDVG.PAD
|A32   DDR1_VTP   OVTPOSHTLTCDVG.PAD
|AT26   HDMI_TMDSDP1   HDMI_PHY.PAD
|AT25   HDMI_TMDSDP0   HDMI_PHY.PAD
|AU26   HDMI_TMDSDN1   HDMI_PHY.PAD
|AU25   HDMI_TMDSDN0   HDMI_PHY.PAD
|AU24   HDMI_TMDSCLKN   HDMI_PHY.PAD
|AT27   HDMI_TMDSDP2   HDMI_PHY.PAD
|AN25   HDMI_EXTSWING   HDMI_PHY.PAD
|AN18   HDMI_CLK_OBS_P   OLVDS18G.PAD
|AT24   HDMI_TMDSCLKP   HDMI_PHY.PAD
|AU27   HDMI_TMDSDN2   HDMI_PHY.PAD
|AN19   HDMI_CLK_OBS_N   OLVDS18G.PADN
|AU37   IFORCE   IPMCSWG.PAD
|AT21   IOUTA   CQ0094.PAD
|AR21   IOUTB   CQ0094.PAD
|AP21   IOUTC   CQ0094.PAD
|AR20   IOUTD   CQ0094.PAD
|AT19   IOUTE   CQ0094.PAD
|AT20   IOUTF   CQ0094.PAD
|AU20   IOUTG   CQ0094.PAD
|AB30   PCIE_TXN0   WIZ7C2B4N5H1PL.PAD
|V30   PCIE_RXN1   WIZ7C2B4N5H1PL.PAD
|V29   PCIE_RXN0   WIZ7C2B4N5H1PL.PAD
|AB36   PCIE_AMUX   WIZ7C2B4N5H1PL.PAD
|V31   PCIE_RXP1   WIZ7C2B4N5H1PL.PAD
|Y29   PCIE_RXP0   WIZ7C2B4N5H1PL.PAD
|AB28   PCIE_TXN1   WIZ7C2B4N5H1PL.PAD
|AB31   PCIE_TXP0   WIZ7C2B4N5H1PL.PAD
|Y27   PCIE_TXP1   WIZ7C2B4N5H1PL.PAD
|N20   PLLOUTN   OCML10G.PADN
|N19   PLLOUTP   OCML10G.PADP
|AU21   RFOUT   CQ0094.PAD
|W35   SATA_RXP1   WIZ7C2B4N5H1PL.PAD
|T31   SATA_TXN0   WIZ7C2B4N5H1PL.PAD
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[Model Selector] Selector_1
Model_411 INPUT,3.3V,PD
Model_412 INPUT,3.3V,PU
Model_413 I/O,3.3V,PI
|   Usage O#1.5V###BSHTLTCSCDVGPBFZ.PAD
|   Base model BSHTLTCSCDVGPBFZ
[Model Selector] Selector_2
Model_100 3-STATE,1.5V,FAST, 8MA,+-5%
Model_101 3-STATE,1.5V,SLOW, 4MA,+-5%
Model_102 3-STATE,1.5V,SLOWEST, 4MA,+-5%
Model_103 3-STATE,1.5V,FASTEST, 6MA,+-5%
Model_104 3-STATE,1.5V,SLOW, 8MA,+-5%
Model_105 3-STATE,1.5V,FASTEST, 10MA,+-5%
Model_106 3-STATE,1.5V,FASTEST, 9MA,+-5%
Model_107 3-STATE,1.5V,FAST, 10MA,+-5%
Model_108 3-STATE,1.5V,SLOWEST, 6MA,+-5%
Model_109 3-STATE,1.5V,FAST, 7MA,+-5%
Model_110 3-STATE,1.5V,SLOW, 10MA,+-5%
Model_111 3-STATE,1.5V,SLOW, 7MA,+-5%
Model_112 3-STATE,1.5V,FAST, 11MA,+-5%
Model_113 3-STATE,1.5V,SLOWEST, 7MA,+-5%
Model_114 3-STATE,1.5V,SLOW, 11MA,+-5%
Model_115 3-STATE,1.5V,FASTEST, 4MA,+-5%
Model_116 3-STATE,1.5V,FASTEST, 8MA,+-5%
Model_117 3-STATE,1.5V,FAST, 6MA,+-5%
Model_118 3-STATE,1.5V,FASTEST, 5MA,+-5%
Model_119 3-STATE,1.5V,FAST, 5MA,+-5%
Model_120 3-STATE,1.5V,SLOW, 6MA,+-5%
Model_121 3-STATE,1.5V,SLOWEST, 8MA,+-5%
Model_122 3-STATE,1.5V,SLOW, 5MA,+-5%
Model_123 3-STATE,1.5V,FASTEST, 7MA,+-5%
Model_124 3-STATE,1.5V,FAST, 9MA,+-5%
Model_125 3-STATE,1.5V,SLOWEST, 5MA,+-5%
Model_126 3-STATE,1.5V,SLOW, 9MA,+-5%
Model_127 3-STATE,1.5V,FASTEST, 11MA,+-5%
Model_128 3-STATE,1.5V,SLOWEST, 10MA,+-5%
Model_129 3-STATE,1.5V,SLOWEST, 9MA,+-5%
Model_34 3-STATE,1.5V,SLOWEST, 11MA,+-10%
Model_35 3-STATE,1.5V,FAST, 4MA,+-10%
Model_36 3-STATE,1.5V,FAST, 8MA,+-10%
Model_37 3-STATE,1.5V,SLOW, 4MA,+-10%
Model_38 3-STATE,1.5V,SLOWEST, 4MA,+-10%
Model_39 3-STATE,1.5V,FASTEST, 6MA,+-10%
Model_40 3-STATE,1.5V,SLOW, 8MA,+-10%
Model_41 3-STATE,1.5V,FASTEST, 10MA,+-10%
Model_42 3-STATE,1.5V,FASTEST, 9MA,+-10%
Model_43 3-STATE,1.5V,FAST, 10MA,+-10%
Model_44 3-STATE,1.5V,SLOWEST, 6MA,+-10%
Model_45 3-STATE,1.5V,FAST, 7MA,+-10%
Model_46 3-STATE,1.5V,SLOW, 10MA,+-10%
Model_47 3-STATE,1.5V,SLOW, 7MA,+-10%
Model_48 3-STATE,1.5V,FAST, 11MA,+-10%
Model_49 3-STATE,1.5V,SLOWEST, 7MA,+-10%
Model_50 3-STATE,1.5V,SLOW, 11MA,+-10%
Model_51 3-STATE,1.5V,FASTEST, 4MA,+-10%
Model_52 3-STATE,1.5V,FASTEST, 8MA,+-10%
Model_53 3-STATE,1.5V,FAST, 6MA,+-10%
Model_54 3-STATE,1.5V,FASTEST, 5MA,+-10%
Model_55 3-STATE,1.5V,FAST, 5MA,+-10%
Model_56 3-STATE,1.5V,SLOW, 6MA,+-10%
Model_57 3-STATE,1.5V,SLOWEST, 8MA,+-10%
Model_58 3-STATE,1.5V,SLOW, 5MA,+-10%
Model_59 3-STATE,1.5V,FASTEST, 7MA,+-10%
Model_60 3-STATE,1.5V,FAST, 9MA,+-10%
Model_61 3-STATE,1.5V,SLOWEST, 5MA,+-10%
Model_62 3-STATE,1.5V,SLOW, 9MA,+-10%
Model_63 3-STATE,1.5V,FASTEST, 11MA,+-10%
Model_64 3-STATE,1.5V,SLOWEST, 10MA,+-10%
Model_65 3-STATE,1.5V,SLOWEST, 9MA,+-10%
Model_98 3-STATE,1.5V,SLOWEST, 11MA,+-5%
Model_99 3-STATE,1.5V,FAST, 4MA,+-5%
|   Usage IO#3.3V#PD/PI/PU##BC3340DGHYPBFBP18.PAD
|   Base model BC3340DGHYPBFBP18
[Model Selector] Selector_3
Model_414 INPUT,3.3V,PD
Model_415 INPUT,3.3V,PU
Model_416 I/O,3.3V,PI
|   Usage IO#1.5V###BSHTLTCSCDVGPBFZ.PAD
|   Base model BSHTLTCSCDVGPBFZ
[Model Selector] Selector_4
Model_100 3-STATE,1.5V,FAST, 8MA,+-5%
Model_101 3-STATE,1.5V,SLOW, 4MA,+-5%
Model_102 3-STATE,1.5V,SLOWEST, 4MA,+-5%
Model_103 3-STATE,1.5V,FASTEST, 6MA,+-5%
Model_104 3-STATE,1.5V,SLOW, 8MA,+-5%
Model_105 3-STATE,1.5V,FASTEST, 10MA,+-5%
Model_106 3-STATE,1.5V,FASTEST, 9MA,+-5%
Model_107 3-STATE,1.5V,FAST, 10MA,+-5%
Model_108 3-STATE,1.5V,SLOWEST, 6MA,+-5%
Model_109 3-STATE,1.5V,FAST, 7MA,+-5%
Model_110 3-STATE,1.5V,SLOW, 10MA,+-5%
Model_111 3-STATE,1.5V,SLOW, 7MA,+-5%
Model_112 3-STATE,1.5V,FAST, 11MA,+-5%
Model_113 3-STATE,1.5V,SLOWEST, 7MA,+-5%
Model_114 3-STATE,1.5V,SLOW, 11MA,+-5%
Model_115 3-STATE,1.5V,FASTEST, 4MA,+-5%
Model_116 3-STATE,1.5V,FASTEST, 8MA,+-5%
Model_117 3-STATE,1.5V,FAST, 6MA,+-5%
Model_118 3-STATE,1.5V,FASTEST, 5MA,+-5%
Model_119 3-STATE,1.5V,FAST, 5MA,+-5%
Model_120 3-STATE,1.5V,SLOW, 6MA,+-5%
Model_121 3-STATE,1.5V,SLOWEST, 8MA,+-5%
Model_122 3-STATE,1.5V,SLOW, 5MA,+-5%
Model_123 3-STATE,1.5V,FASTEST, 7MA,+-5%
Model_124 3-STATE,1.5V,FAST, 9MA,+-5%
Model_125 3-STATE,1.5V,SLOWEST, 5MA,+-5%
Model_126 3-STATE,1.5V,SLOW, 9MA,+-5%
Model_127 3-STATE,1.5V,FASTEST, 11MA,+-5%
Model_128 3-STATE,1.5V,SLOWEST, 10MA,+-5%
Model_129 3-STATE,1.5V,SLOWEST, 9MA,+-5%
Model_133 INPUT,1.5V,HALFTERM,+-10%
Model_134 INPUT,1.5V,NOTERM,+-10%
Model_135 INPUT,1.5V,FULLTERM,+-10%
Model_139 INPUT,1.5V,HALFTERM,+-5%
Model_140 INPUT,1.5V,NOTERM,+-5%
Model_141 INPUT,1.5V,FULLTERM,+-5%
Model_34 3-STATE,1.5V,SLOWEST, 11MA,+-10%
Model_35 3-STATE,1.5V,FAST, 4MA,+-10%
Model_36 3-STATE,1.5V,FAST, 8MA,+-10%
Model_37 3-STATE,1.5V,SLOW, 4MA,+-10%
Model_38 3-STATE,1.5V,SLOWEST, 4MA,+-10%
Model_39 3-STATE,1.5V,FASTEST, 6MA,+-10%
Model_40 3-STATE,1.5V,SLOW, 8MA,+-10%
Model_41 3-STATE,1.5V,FASTEST, 10MA,+-10%
Model_42 3-STATE,1.5V,FASTEST, 9MA,+-10%
Model_43 3-STATE,1.5V,FAST, 10MA,+-10%
Model_44 3-STATE,1.5V,SLOWEST, 6MA,+-10%
Model_45 3-STATE,1.5V,FAST, 7MA,+-10%
Model_46 3-STATE,1.5V,SLOW, 10MA,+-10%
Model_47 3-STATE,1.5V,SLOW, 7MA,+-10%
Model_48 3-STATE,1.5V,FAST, 11MA,+-10%
Model_49 3-STATE,1.5V,SLOWEST, 7MA,+-10%
Model_50 3-STATE,1.5V,SLOW, 11MA,+-10%
Model_51 3-STATE,1.5V,FASTEST, 4MA,+-10%
Model_52 3-STATE,1.5V,FASTEST, 8MA,+-10%
Model_53 3-STATE,1.5V,FAST, 6MA,+-10%
Model_54 3-STATE,1.5V,FASTEST, 5MA,+-10%
Model_55 3-STATE,1.5V,FAST, 5MA,+-10%
Model_56 3-STATE,1.5V,SLOW, 6MA,+-10%
Model_57 3-STATE,1.5V,SLOWEST, 8MA,+-10%
Model_58 3-STATE,1.5V,SLOW, 5MA,+-10%
Model_59 3-STATE,1.5V,FASTEST, 7MA,+-10%
Model_60 3-STATE,1.5V,FAST, 9MA,+-10%
Model_61 3-STATE,1.5V,SLOWEST, 5MA,+-10%
Model_62 3-STATE,1.5V,SLOW, 9MA,+-10%
Model_63 3-STATE,1.5V,FASTEST, 11MA,+-10%
Model_64 3-STATE,1.5V,SLOWEST, 10MA,+-10%
Model_65 3-STATE,1.5V,SLOWEST, 9MA,+-10%
Model_98 3-STATE,1.5V,SLOWEST, 11MA,+-5%
Model_99 3-STATE,1.5V,FAST, 4MA,+-5%
|   Usage IO#3.3V###BI2C33GFZP18.PAD
|   Base model BI2C33GFZP18
[Model Selector] Selector_5
Model_410 I/O_OPEN_DRAIN,3.3V
|   Usage O#3.3V#PD/PI/PU##BC3340CGHYPBFBP18.PAD
|   Base model BC3340CGHYPBFBP18
[Model Selector] Selector_6
Model_413 I/O,3.3V,PI
|   Usage IO#1.5V###BSHTLTCSCDDVGPBFZ.*
|   Base model BSHTLTCSCDDVGPBFZ
[Model Selector] Selector_7
Model_174 3-STATE,1.5V,SLOWEST, 11MA,+-10%
Model_175 3-STATE,1.5V,FAST, 4MA,+-10%
Model_176 3-STATE,1.5V,FAST, 8MA,+-10%
Model_177 3-STATE,1.5V,SLOW, 4MA,+-10%
Model_178 3-STATE,1.5V,SLOWEST, 4MA,+-10%
Model_179 3-STATE,1.5V,FASTEST, 6MA,+-10%
Model_180 3-STATE,1.5V,SLOW, 8MA,+-10%
Model_181 3-STATE,1.5V,FASTEST, 10MA,+-10%
Model_182 3-STATE,1.5V,FASTEST, 9MA,+-10%
Model_183 3-STATE,1.5V,FAST, 10MA,+-10%
Model_184 3-STATE,1.5V,SLOWEST, 6MA,+-10%
Model_185 3-STATE,1.5V,FAST, 7MA,+-10%
Model_186 3-STATE,1.5V,SLOW, 10MA,+-10%
Model_187 3-STATE,1.5V,SLOW, 7MA,+-10%
Model_188 3-STATE,1.5V,FAST, 11MA,+-10%
Model_189 3-STATE,1.5V,SLOWEST, 7MA,+-10%
Model_190 3-STATE,1.5V,SLOW, 11MA,+-10%
Model_191 3-STATE,1.5V,FASTEST, 4MA,+-10%
Model_192 3-STATE,1.5V,FASTEST, 8MA,+-10%
Model_193 3-STATE,1.5V,FAST, 6MA,+-10%
Model_194 3-STATE,1.5V,FASTEST, 5MA,+-10%
Model_195 3-STATE,1.5V,FAST, 5MA,+-10%
Model_196 3-STATE,1.5V,SLOW, 6MA,+-10%
Model_197 3-STATE,1.5V,SLOWEST, 8MA,+-10%
Model_198 3-STATE,1.5V,SLOW, 5MA,+-10%
Model_199 3-STATE,1.5V,FASTEST, 7MA,+-10%
Model_200 3-STATE,1.5V,FAST, 9MA,+-10%
Model_201 3-STATE,1.5V,SLOWEST, 5MA,+-10%
Model_202 3-STATE,1.5V,SLOW, 9MA,+-10%
Model_203 3-STATE,1.5V,FASTEST, 11MA,+-10%
Model_204 3-STATE,1.5V,SLOWEST, 10MA,+-10%
Model_205 3-STATE,1.5V,SLOWEST, 9MA,+-10%
Model_238 3-STATE,1.5V,SLOWEST, 11MA,+-5%
Model_239 3-STATE,1.5V,FAST, 4MA,+-5%
Model_240 3-STATE,1.5V,FAST, 8MA,+-5%
Model_241 3-STATE,1.5V,SLOW, 4MA,+-5%
Model_242 3-STATE,1.5V,SLOWEST, 4MA,+-5%
Model_243 3-STATE,1.5V,FASTEST, 6MA,+-5%
Model_244 3-STATE,1.5V,SLOW, 8MA,+-5%
Model_245 3-STATE,1.5V,FASTEST, 10MA,+-5%
Model_246 3-STATE,1.5V,FASTEST, 9MA,+-5%
Model_247 3-STATE,1.5V,FAST, 10MA,+-5%
Model_248 3-STATE,1.5V,SLOWEST, 6MA,+-5%
Model_249 3-STATE,1.5V,FAST, 7MA,+-5%
Model_250 3-STATE,1.5V,SLOW, 10MA,+-5%
Model_251 3-STATE,1.5V,SLOW, 7MA,+-5%
Model_252 3-STATE,1.5V,FAST. 11MA,+-5%
Model_253 3-STATE,1.5V,SLOWEST, 7MA,+-5%
Model_254 3-STATE,1.5V,SLOW, 11MA,+-5%
Model_255 3-STATE,1.5V,FASTEST, 4MA,+-5%
Model_256 3-STATE,1.5V,FASTEST, 8MA,+-5%
Model_257 3-STATE,1.5V,FAST, 6MA,+-5%
Model_258 3-STATE,1.5V,FASTEST, 6MA,+-5%
Model_259 3-STATE,1.5V,FAST, 5MA,+-5%
Model_260 3-STATE,1.5V,SLOW, 6MA,+-5%
Model_261 3-STATE,1.5V,SLOWEST, 8MA,+-5%
Model_262 3-STATE,1.5V,SLOW, 5MA,+-5%
Model_263 3-STATE,1.5V,FASTEST, 7MA,+-5%
Model_264 3-STATE,1.5V,FAST, 8MA,+-5%
Model_265 3-STATE,1.5V,SLOWEST, 5MA,+-5%
Model_266 3-STATE,1.5V,SLOW, 9MA,+-5%
Model_267 3-STATE,1.5V,FASTEST, 11MA,+-5%
Model_268 3-STATE,1.5V,SLOWEST, 10MA,+-5%
Model_269 3-STATE,1.5V,SLOWEST, 9MA,+-5%
Model_302 3-STATE,1.5V,SLOWEST, 11MA,+-10%
Model_303 3-STATE,1.5V,FAST, 4MA,+-10%
Model_304 3-STATE,1.5V,FAST, 8MA,+-10%
Model_305 3-STATE,1.5V,SLOW, 4MA,+-10%
Model_306 3-STATE,1.5V,SLOWEST, 4MA,+-10%
Model_307 3-STATE,1.5V,FASTEST, 6MA,+-10%
Model_308 3-STATE,1.5V,SLOW, 8MA,+-10%
Model_309 3-STATE,1.5V,FASTEST, 10MA,+-10%
Model_310 3-STATE,1.5V,FASTEST, 9MA,+-10%
Model_311 3-STATE,1.5V,FAST, 10MA,+-10%
Model_312 3-STATE,1.5V,SLOWEST, 6MA,+-10%
Model_313 3-STATE,1.5V,FAST, 7MA,+-10%
Model_314 3-STATE,1.5V,SLOW, 10MA,+-10%
Model_315 3-STATE,1.5V,SLOW, 7MA,+-10%
Model_316 3-STATE,1.5V,FAST, 11MA,+-10%
Model_317 3-STATE,1.5V,SLOWEST, 7MA,+-10%
Model_318 3-STATE,1.5V,SLOW, 11MA,+-10%
Model_319 3-STATE,1.5V,FASTEST, 4MA,+-10%
Model_320 3-STATE,1.5V,FASTEST, 8MA,+-10%
Model_321 3-STATE,1.5V,FAST, 6MA,+-10%
Model_322 3-STATE,1.5V,FASTEST, 5MA,+-10%
Model_323 3-STATE,1.5V,FAST, 5MA,+-10%
Model_324 3-STATE,1.5V,SLOW, 6MA,+-10%
Model_325 3-STATE,1.5V,SLOWEST, 8MA,+-10%
Model_326 3-STATE,1.5V,SLOW, 5MA,+-10%
Model_327 3-STATE,1.5V,FASTEST, 7MA,+-10%
Model_328 3-STATE,1.5V,FAST, 9MA,+-10%
Model_329 3-STATE,1.5V,SLOWEST, 5MA,+-10%
Model_330 3-STATE,1.5V,SLOW, 9MA,+-10%
Model_331 3-STATE,1.5V,FASTEST, 11MA,+-10%
Model_332 3-STATE,1.5V,SLOWEST, 10MA,+-10%
Model_333 3-STATE,1.5V,SLOWEST, 9MA,+-10%
Model_366 3-STATE,1.5V,SLOWEST, 11MA,+-5%
Model_367 3-STATE,1.5V,FAST, 4MA,+-5%
Model_368 3-STATE,1.5V,FAST, 8MA,+-5%
Model_369 3-STATE,1.5V,SLOW, 4MA,+-5%
Model_370 3-STATE,1.5V,SLOWEST, 4MA,+-5%
Model_371 3-STATE,1.5V,FASTEST, 6MA,+-5%
Model_372 3-STATE,1.5V,SLOW, 8MA,+-5%
Model_373 3-STATE,1.5V,FASTEST, 10MA,+-5%
Model_374 3-STATE,1.5V,FASTEST, 9MA,+-5%
Model_375 3-STATE,1.5V,FAST, 10MA,+-5%
Model_376 3-STATE,1.5V,SLOWEST, 6MA,+-5%
Model_377 3-STATE,1.5V,FAST, 7MA,+-5%
Model_378 3-STATE,1.5V,SLOW, 10MA,+-5%
Model_379 3-STATE,1.5V,SLOQ, 7MA,+-5%
Model_380 3-STATE,1.5V,FAST, 11MA,+-5%
Model_381 3-STATE,1.5V,SLOWEST, 7MA,+-5%
Model_382 3-STATE,1.5V,SLOW, 11MA,+-5%
Model_383 3-STATE,1.5V,FASTEST, 4MA,+-5%
Model_384 3-STATE,1.5V,FASTEST, 8MA,+-5%
Model_385 3-STATE,1.5V,FAST, 6MA,+-5%
Model_386 3-STATE,1.5V,FASTEST, 5MA,+-5%
Model_387 3-STATE,1.5V,FAST, 5MA,+-5%
Model_388 3-STATE,1.5V,SLOW, 6MA,+-5%
Model_389 3-STATE,1.5V,SLOWEST, 8MA,+-5%
Model_390 3-STATE,1.5V,SLOW, 5MA,+-5%
Model_391 3-STATE,1.5V,FASTEST, 7MA,+-5%
Model_392 3-STATE,1.5V,FAST, 9MA,+-5%
Model_393 3-STATE,1.5V,SLOWEST, 5MA,+-5%
Model_394 3-STATE,1.5V,SLOW, 9MA,+-5%
Model_395 3-STATE,1.5V,FASTEST, 11MA,+-5%
Model_396 3-STATE,1.5V,SLOWEST, 10MA,+-5%
Model_397 3-STATE,1.5V,SLOWEST, 9MA,+-5%
Model_401 INPUT,1.5V,HALFTERM,+-10%
Model_402 INPUT,1.5V,NOTERM,+-10%
Model_403 INPUT,1.5V,FULLTERM,+-10%
Model_407 INPUT,1.5V,HALFTERM,+-5%
Model_408 INPUT,1.5V,NOTERM,+-5%
Model_409 INPUT,1.5V,FULLTERM,+-5%
|   Usage I#3.3V#PD/PI/PU##IQ33GHYPBFBP18.PAD
|   Base model IQ33GHYPBFBP18
[Model Selector] Selector_8
Model_417 INPUT,3.3V,PD
Model_418 INPUT,3.3V,PU
Model_419 INPUT,3.3V,PI
|   Usage I#3.3V###IHHV33GP18.PAD
|   Base model IHHV33GP18
[Model Selector] Selector_9
Model_1 INPUT,3.3V
| Models and submodels in the file (215): Model_1 (Input), Model_34 (3-state), Model_35 (3-state), Model_36 (3-state), Model_37 (3-state), Model_38 (3-state), Model_39 (3-state), Model_40 (3-state), Model_41 (3-state), Model_42 (3-state), Model_43 (3-state), Model_44 (3-state), Model_45 (3-state), Model_46 (3-state), Model_47 (3-state), Model_48 (3-state), Model_49 (3-state), Model_50 (3-state), Model_51 (3-state), Model_52 (3-state), Model_53 (3-state), Model_54 (3-state), Model_55 (3-state), Model_56 (3-state), Model_57 (3-state), Model_58 (3-state), Model_59 (3-state), Model_60 (3-state), Model_61 (3-state), Model_62 (3-state), Model_63 (3-state), Model_64 (3-state), Model_65 (3-state), Model_98 (3-state), Model_99 (3-state), Model_100 (3-state), Model_101 (3-state), Model_102 (3-state), Model_103 (3-state), Model_104 (3-state), Model_105 (3-state), Model_106 (3-state), Model_107 (3-state), Model_108 (3-state), Model_109 (3-state), Model_110 (3-state), Model_111 (3-state), Model_112 (3-state), Model_113 (3-state), Model_114 (3-state), Model_115 (3-state), Model_116 (3-state), Model_117 (3-state), Model_118 (3-state), Model_119 (3-state), Model_120 (3-state), Model_121 (3-state), Model_122 (3-state), Model_123 (3-state), Model_124 (3-state), Model_125 (3-state), Model_126 (3-state), Model_127 (3-state), Model_128 (3-state), Model_129 (3-state), Model_133 (Input), Model_134 (Input), Model_135 (Input), Model_139 (Input), Model_140 (Input), Model_141 (Input), Model_174 (3-state), Model_175 (3-state), Model_176 (3-state), Model_177 (3-state), Model_178 (3-state), Model_179 (3-state), Model_180 (3-state), Model_181 (3-state), Model_182 (3-state)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
